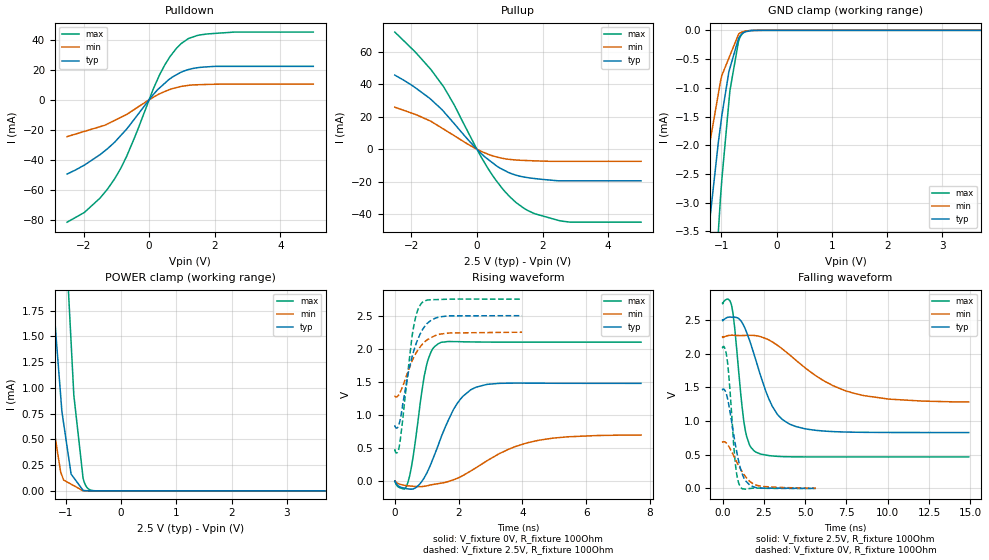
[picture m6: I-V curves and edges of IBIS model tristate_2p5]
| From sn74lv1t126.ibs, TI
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|   tristate_2p5 Model
[Model]   tristate_2p5
Model_type   3-state
Polarity   Non-Inverting
Vmeas = 1.25
Vref = 0
Cref = 30pF
Rref = 200
|   typ   min   max
|   (nom PVT)   (fast PVT)   (slow PVT)
C_comp   2.155e-12   2.082e-12   2.233e-12
| Where nom  PVT is Nominal Process, 2.5V, 40C
|   Fast PVT is Strong Process,  2.75V, -40C
|   Slow PVT is Weak Process,   2.25V, 140C
[Voltage Range]   2.5   2.25   2.75
|Junction Temperature
[Temperature Range]   40   140   -40
[Pullup Reference]   2.5   2.25   2.75
[Pulldown Reference]   0   0   0
[Power Clamp Reference]   2.5   2.25   2.75
[GND Clamp Reference]   0   0   0
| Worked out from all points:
|   slope of the pulldown table from 0 to 0.375 V, typ, clamps not added: 41.7 ohm
|   slope of the pullup table from 0 to 0.375 V, typ, clamps not added: 55.3 ohm
|   GND clamp passes 1 mA (typ) near -0.91 V on its own axis
|   POWER clamp passes 1 mA (typ) near -1.10 V on its own axis
|   falling waveform, V_fixture 2.5V, R_fixture 100Ohm: 20-80 % time 1.48ns typ, 3.47ns min, 565ps max; typ from 2.5 V to 0.829 V
|   rising waveform, V_fixture 0V, R_fixture 100Ohm: 20-80 % time 810ps typ, 1.68ns min, 373ps max; typ from 0 V to 1.48 V
|   rising waveform, V_fixture 2.5V, R_fixture 100Ohm: 20-80 % time 493ps typ, 563ps min, 329ps max; typ from 0.829 V to 2.5 V
|   falling waveform, V_fixture 0V, R_fixture 100Ohm: 20-80 % time 667ps typ, 970ps min, 378ps max; typ from 1.48 V to 0.001 V
[Pulldown]
|   Voltage   I(typ)   I(min)   I(max)
-2.5V     -49.51mA   -24.58mA   -81.56mA
-1.977V   -43.59mA   -21.13mA   -75.13mA
-1.49V    -36.5mA    -17.92mA   -65.38mA
-1.053V   -28.34mA   -13.78mA   -52.74mA
-687.5mV  -19.61mA   -9.851mA   -37.79mA
115.5mV   3.133mA    1.469mA    6.581mA
319mV     7.9mA      3.952mA    16.65mA
640.8mV   14.06mA    6.881mA    28.89mA
990mV     18.48mA    8.91mA     37.63mA
1.216V    20.2mA     9.611mA    40.93mA
1.774V    21.9mA     10.18mA    43.81mA
5V        22.22mA    10.36mA    45.04mA
[GND Clamp]
|   Voltage   I(typ)   I(min)   I(max)
-2.5V     -22.56mA   -12.71mA   -37.03mA
-1.485V   -6.342mA   -3.663mA   -11.17mA
-1.425V   -5.659mA   -3.245mA   -9.918mA
-1.361V   -4.945mA   -2.809mA   -8.659mA
-1.21V    -3.314mA   -1.971mA   -5.887mA
-1.052V   -1.941mA   -1.097mA   -3.487mA
-990mV    -1.481mA   -784.7uA   -2.592mA
-844.2mV  -657.8uA   -438.7uA   -1.05mA
-687.5mV  -137.7uA   -66.69uA   -185.2uA
-634.5mV  -67.99uA   -33.81uA   -79.05uA
-451mV    -3.555uA   -3.759uA   -2.087uA
5V        0A         0A         0A
[Pullup]
|   Voltage   I(typ)   I(min)   I(max)
-2.5V     45.52mA    25.81mA    71.95mA
-1.881V   37.86mA    21.44mA    59.82mA
-1.403V   30.64mA    17.18mA    49mA
-1.006V   23.02mA    12.25mA    38.16mA
-687.5mV  15.64mA    8.29mA     27.11mA
-217.5mV  4.704mA    2.429mA    8.492mA
349.3mV   -6.378mA   -3.133mA   -12.17mA
775.5mV   -12.35mA   -5.563mA   -24.15mA
1.199V    -15.98mA   -6.635mA   -32.86mA
1.774V    -18.04mA   -7.15mA    -39.69mA
2.596V    -19.39mA   -7.423mA   -44.19mA
5V        -19.39mA   -7.423mA   -44.82mA
[POWER Clamp]
|   Voltage   I(typ)   I(min)   I(max)
-2.5V     19.77mA    9.741mA    37.38mA
-1.7V     6.773mA    3.06mA     15.28mA
-1.495V   4.296mA    1.749mA    10.75mA
-1.402V   3.37mA     1.231mA    8.88mA
-1.243V   1.954mA    691.3uA    5.896mA
-1.093V   924.1uA    182.9uA    3.605mA
-1.037V   644.8uA    104.7uA    2.813mA
-905mV    163.5uA    65.67uA    1.445mA
-855.2mV  127.3uA    50.94uA    928.1uA
-686.3mV  5.211uA    897.5nA    119.4uA
-453.7mV  70.98nA    33.3nA     971.7nA
5V        0A         0A         0A
[Ramp]
R_load = 100
|   typ   min   max
dV/dt_r   0.886983/8.08573e-10  0.418962/1.6671e-09   1.26024/3.70773e-10
dV/dt_f   1.00241/1.46185e-09   0.583073/3.49087e-09   1.36941/5.63248e-10
[Falling Waveform]
V_fixture = 2.5V
V_fixture_min = 2.25V
V_fixture_max = 2.75V
R_fixture = 100Ohm
|   Time   V(typ)   V(min)   V(max)
0s        2.5V       2.25V      2.75V
544ps     2.539V     2.272V     2.716V
726ps     2.54V      2.271V     2.4V
1.338ns   2.386V     2.269V     916.1mV
1.634ns   2.196V     2.271V     645.1mV
2.016ns   1.902V     2.266V     538.6mV
3.026ns   1.212V     2.171V     481.9mV
4.416ns   920.3mV    1.907V     468.6mV
7.904ns   834.6mV    1.414V     467.6mV
14.91ns   829.3mV    1.283V     467.6mV
[Rising Waveform]
V_fixture = 0V
V_fixture_min = 0V
V_fixture_max = 0V
R_fixture = 100Ohm
|   Time   V(typ)   V(min)   V(max)
0s        620.8pV    12.98nV    744.7pV
300ps     -105.6mV   -61.99mV   -120.3mV
408ps     -115.7mV   -68.99mV   -23.3mV
570ps     -117.6mV   -76.27mV   357.5mV
988ps     109.1mV    -71.78mV   1.738V
1.348ns   526.4mV    -37.94mV   2.072V
1.954ns   1.172V     42.65mV    2.109V
2.548ns   1.42V      203.1mV    2.103V
4.524ns   1.481V     619.2mV    2.1V
7.724ns   1.478V     697.3mV    2.1V
[Rising Waveform]
V_fixture = 2.5V
V_fixture_min = 2.25V
V_fixture_max = 2.75V
R_fixture = 100Ohm
|   Time   V(typ)   V(min)   V(max)
0s        829.3mV    1.278V     467.6mV
82ps      808.3mV    1.281V     435.3mV
156ps     903.7mV    1.332V     571.9mV
394ps     1.57V      1.631V     1.579V
580ps     1.946V     1.858V     2.306V
708ps     2.128V     1.97V      2.57V
848ps     2.273V     2.06V      2.694V
1.144ns   2.433V     2.17V      2.741V
1.41ns    2.482V     2.221V     2.745V
3.99ns    2.5V       2.25V      2.75V
[Falling Waveform]
V_fixture = 0V
V_fixture_min = 0V
V_fixture_max = 0V
R_fixture = 100Ohm
|   Time   V(typ)   V(min)   V(max)
0s        1.478V     698.3mV    2.1V
158ps     1.447V     687.3mV    2.066V
298ps     1.337V     653.1mV    1.875V
438ps     1.155V     599.1mV    1.491V
762ps     670.2mV    439.8mV    400mV
898ps     492.5mV    373mV      157.1mV
1.056ns   321.5mV    301mV      34.27mV
1.41ns    109.4mV    168.4mV    -10.38mV
1.98ns    15.8mV     55.62mV    5.027mV
5.646ns   853.1uV    5.468mV    -2.969uV
